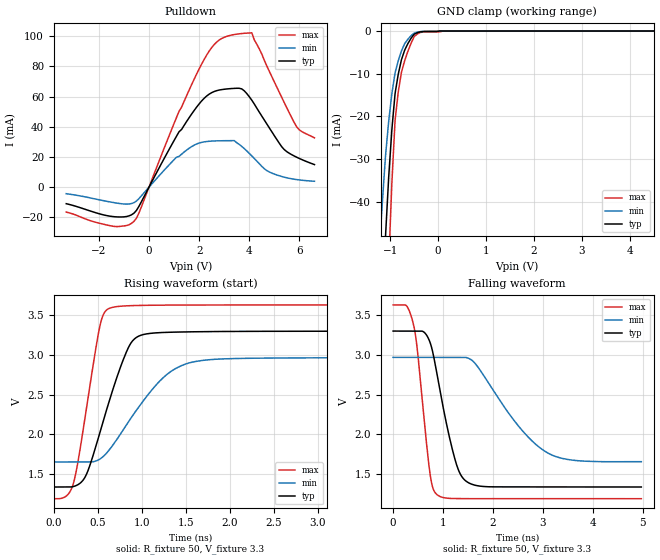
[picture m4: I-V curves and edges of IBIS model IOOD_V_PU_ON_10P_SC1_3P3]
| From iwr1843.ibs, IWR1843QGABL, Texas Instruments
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|   Model Cell IOOD_V_PU_ON_10P_SC1_3P3
|IOOD_V_PU_ON_10P_SC1_3P3
[Model]   IOOD_V_PU_ON_10P_SC1_3P3
Model_type   I/O_open_drain
Polarity   Non-Inverting
Enable   Active-Low
Vinl =  0.8V
Vinh =  2V
Cref =  15pF
Rref =  100.0000M
Vref =  0V
Vmeas =  1.65
|   typ   min   max
C_comp   2.059994p   1.912853p   2.135747p
[Model Spec]
Vinl   0.8V   0.8V   0.8V
Vinh   2V   2V   2V
[Temperature Range]   25   125   -40
[Voltage Range]   3.3   2.97   3.63
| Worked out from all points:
|   slope of the pulldown table from 0 to 0.495 V, typ, clamps not added: 31.8 ohm
|   GND clamp passes 1 mA (typ) near -0.52 V on its own axis
|   rising waveform, R_fixture 50, V_fixture 3.3: 20-80 % time 333ps typ, 531ps min, 208ps max; typ from 1.34 V to 3.3 V
|   falling waveform, R_fixture 50, V_fixture 3.3: 20-80 % time 385ps typ, 931ps min, 233ps max; typ from 3.3 V to 1.34 V
| Where Nom  PVT is Nominal Process, 3.3V, 25C
|   Fast PVT is Strong Process,  3.63V, -40C
|   Slow PVT is Weak Process,   2.97V, 125C
[Pulldown]
|   voltage   I(typ)   I(min)   I(max)
-3.3V     -10.93mA   -4.311mA   -16.48mA
-1.4V     -19.53mA   -10.23mA   -25.96mA
-600mV    -17.23mA   -10.26mA   -22.66mA
1.1V      33.82mA    19.89mA    46.25mA
2V        55.14mA    29.24mA    78.29mA
2.6V      63.35mA    30.61mA    94.45mA
3.2V      65.21mA    30.81mA    100.4mA
3.7V      65.09mA    27.02mA    101.8mA
4.1V      57.63mA    20.71mA    102.2mA
5.3V      26.68mA    7.058mA    59.31mA
5.9V      19.77mA    5.007mA    39.76mA
6.6V      14.97mA    3.923mA    32.7mA
[GND_clamp]
|   voltage   I(typ)   I(min)   I(max)
-3.3V     -787.2mA   -607.8mA   -1.235A
-1.233V   -85.67mA   -52.14mA   -138.8mA
-1.167V   -66.48mA   -40.37mA   -107.8mA
-1.1V     -48.26mA   -29.37mA   -78.02mA
-1.033V   -34.3mA    -21.2mA    -54.63mA
-966.7mV  -23.1mA    -14.67mA   -35.61mA
-900mV    -14.66mA   -9.802mA   -20.96mA
-833.3mV  -10.12mA   -6.954mA   -14.3mA
-700mV    -4.501mA   -2.964mA   -6.982mA
-500mV    -717.7uA   -486.4uA   -1.28mA
100mV     0A         0A         0A
6.6V      0A         0A         0A
[Ramp]
| variable   typ   min   max
dV/dt_f  1.1795005/0.38538156n 0.79412542/0.93863952n  1.4659129/0.23394861n
dV/dt_r  1.1738038/0.46664111n 0.80280986/1.0806094n  1.4758979/0.24442591n
R_load = 50
[Rising Waveform]
R_fixture = 50
V_fixture = 3.3
V_fixture_min = 2.97
V_fixture_max = 3.63
|   time   V(typ)   V(min)   V(max)
0s        1.338V     1.653V     1.191V
223.4ps   1.344V     1.653V     1.387V
365.8ps   1.486V     1.653V     2.289V
518.6ps   2.003V     1.686V     3.336V
629.4ps   2.417V     1.804V     3.586V
811.6ps   3.001V     2.095V     3.618V
922.1ps   3.207V     2.278V     3.622V
1.255ns   3.284V     2.726V     3.627V
1.553ns   3.291V     2.904V     3.628V
4.974ns   3.3V       2.968V     3.63V
[Falling Waveform]
R_fixture = 50
V_fixture = 3.3
V_fixture_min = 2.97
V_fixture_max = 3.63
|   time   V(typ)   V(min)   V(max)
0s        3.3V       2.969V     3.629V
269.8ps   3.3V       2.969V     3.617V
406ps     3.3V       2.969V     3.388V
482.4ps   3.3V       2.969V     3.083V
737.7ps   3.161V     2.969V     1.514V
887.2ps   2.732V     2.969V     1.238V
1.254ns   1.654V     2.969V     1.192V
1.51ns    1.391V     2.958V     1.191V
3.071ns   1.338V     1.776V     1.19V
4.974ns   1.338V     1.656V     1.19V
